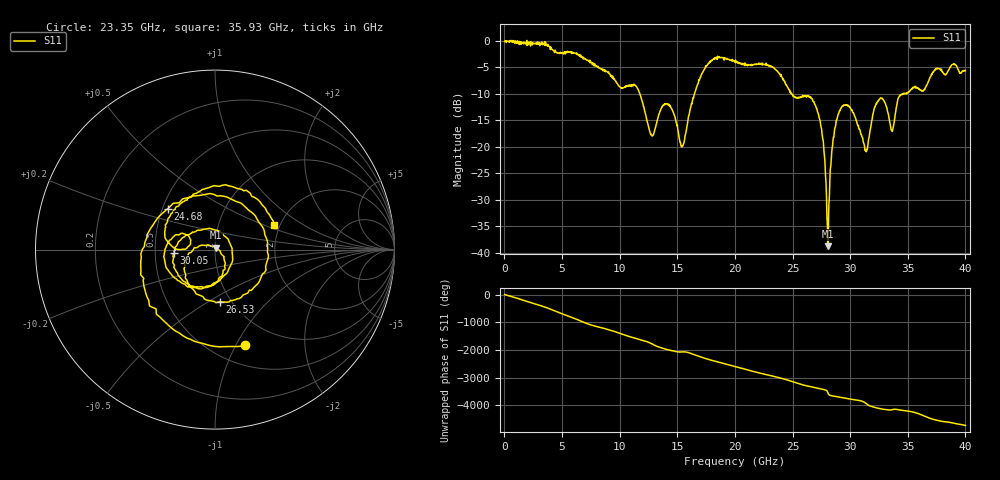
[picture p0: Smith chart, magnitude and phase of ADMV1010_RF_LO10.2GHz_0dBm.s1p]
! Analog Devices, Inc.
! 1 Analog Way
! Wilmington, MA 01887
! http://www.analog.com
! Date:  2021-09-07 NN
! Board Name:  ADMV1010-EVALZ Revision B with ADMV1010AEZ installed
! File Description:  S-Parameters for evaluation board without connectors or board loss de-embedded
! File Generation:  Calibrated Network Analyzer
! Chip Part Number:  ADMV1010
! Chip Description:  GaAs, MMIC, IQ Downconverter
! Chip Frequency:  12.6 to 15.4 GHz
! Chip Package:  LCC, 4.9 x 4.9 x 1 mm
! Chip State:
!  Temperature:  25C
!  LO Frequency:  10.2GHz
!  LO Power:  0dBm
! Note:
!  Analog Devices supplies this data as a sample of measured data at the evaluation board
!  ports for this product.  Your particular data for this product may vary.
!  Analog Devices reserves the right to change this data at anytime.
!  All lines below in this file are as is from the Network Analyzer.
!Keysight Technologies,N5245A,MY49151104,A.10.65.16
!Date: Thursday, August 05, 2021 16:35:58
!Correction: S11(Full 2 Port(1,2))
!S1P File: Measurement: S11:
# Hz S  dB  R 50
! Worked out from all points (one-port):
!   1601 points, 10 MHz to 40 GHz, reference 50 ohm
!   lowest |S11| = -38.8 dB at 28.05 GHz (marker M1), VSWR 1.02, Z = 50.3 + j1.11 ohm
!   |S11| at or under -10 dB: 11.75 GHz to 16.48 GHz (4.726 GHz wide, 33.5 % of centre); 24.91 GHz to 34.53 GHz (9.617 GHz wide, 32.4 % of centre); 34.52654 GHz to 34.58877 GHz (62.23 MHz wide, 0.18 % of centre)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
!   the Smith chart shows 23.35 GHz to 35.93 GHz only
!   S11 on the Smith chart (normalised r, x): 23.35 GHz: 0.71, -1.09; 24.68 GHz: 0.53, +0.28; 26.53 GHz: 0.89, -0.56; 30.05 GHz: 0.63, -0.03; 35.93 GHz: 1.86, +0.58
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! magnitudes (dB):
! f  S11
! 10 MHz  -0.1
! 5.009 GHz  -2.3
! 10.01 GHz  -8.7
! 11.48 GHz  -8.7
! 12.76 GHz  -17.8
! 13.98 GHz  -11.8
! 15.01 GHz  -15.9
! 15.51 GHz  -19.6
! 16.53 GHz  -9.7
! 17.66 GHz  -4.4
! 20 GHz  -4.0
! 23.35 GHz  -5.1
! 24.68 GHz  -9.2
! 25 GHz  -10.1
! 26.53 GHz  -10.7
! 27.48 GHz  -16.3
! 28.05 GHz  -38.8
! 28.83 GHz  -14.9
! 30 GHz  -12.6
! 30.05 GHz  -12.8
! 31.35 GHz  -20.6
! 32.45 GHz  -11.3
! 33.63 GHz  -17.0
! 34.25 GHz  -10.5
! 35 GHz  -9.8
! 35.93 GHz  -9.0
! 37.53 GHz  -5.3
! 40 GHz  -5.6
